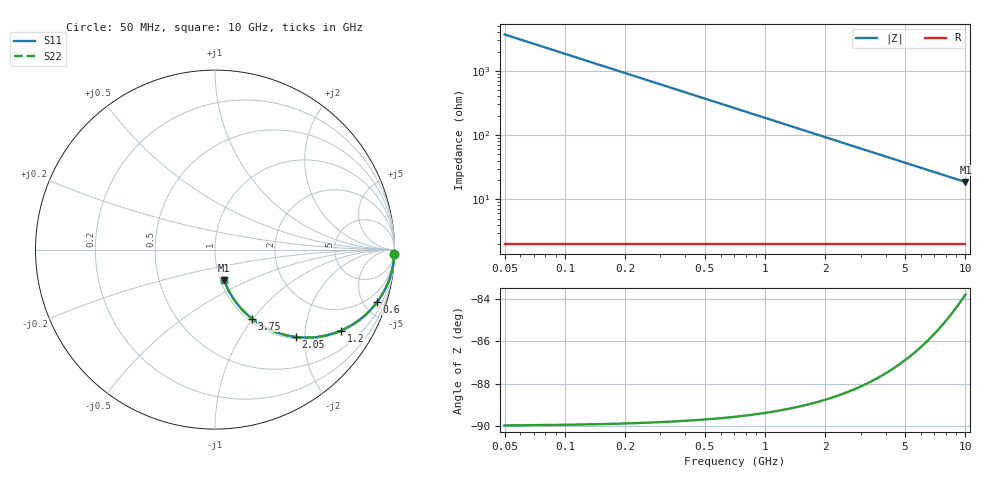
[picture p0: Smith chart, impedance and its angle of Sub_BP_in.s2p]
! Created Thu Jul 12 14:06:35 2018
# hz S ma R 50
! 2 Port Network Data from SP1.SP block
! freq  magS11  angS11  magS21  angS21  magS12  angS12  magS22  angS22
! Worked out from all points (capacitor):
!   200 points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, 50 MHz to 10 GHz, reference 50 ohm
!   read as one part in series: C = 861 fF near 100 MHz
!   lowest |Z| = 18.6 ohm at 10 GHz (marker M1)
!   S11 on the Smith chart (normalised r, x): 50 MHz: 1, -74; 600 MHz: 1.04, -6.16; 1.2 GHz: 1.04, -3.08; 2.05 GHz: 1.04, -1.80; 3.75 GHz: 1.04, -0.99; 10 GHz: 1.04, -0.37
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5e7  0.9996 -1.5  0.02704 88.4  0.02704 88.4  0.9996 -1.5
1e8  0.9985 -3.1  0.05403 86.8  0.05403 86.8  0.9985 -3.1
1.5e8  0.9966 -4.6  0.08089 85.3  0.08089 85.3  0.9966 -4.6
2e8  0.994 -6.2  0.1076 83.7  0.1076 83.7  0.994 -6.2
2.5e8  0.9906 -7.7  0.134 82.1  0.134 82.1  0.9906 -7.7
3.5e8  0.9819 -10.7  0.1859 79.1  0.1859 79.1  0.9819 -10.7
4.5e8  0.9705 -13.7  0.2363 76.1  0.2363 76.1  0.9705 -13.7
6e8  0.9493 -18.0  0.3082 71.7  0.3082 71.7  0.9493 -18.0
7e8  0.9328 -20.7  0.3533 68.9  0.3533 68.9  0.9328 -20.7
8.5e8  0.9053 -24.6  0.4164 64.9  0.4164 64.9  0.9053 -24.6
1e9  0.8755 -28.3  0.4737 61.1  0.4737 61.1  0.8755 -28.3
1.2e9  0.8338 -32.8  0.5413 56.5  0.5413 56.5  0.8338 -32.8
1.45e9  0.7808 -37.8  0.6125 51.3  0.6125 51.3  0.7808 -37.8
1.75e9  0.7194 -42.9  0.6811 46.0  0.6811 46.0  0.7194 -42.9
2.05e9  0.6624 -47.3  0.7345 41.5  0.7345 41.5  0.6624 -47.3
2.7e9  0.5574 -54.5  0.814 33.9  0.814 33.9  0.5574 -54.5
3.4e9  0.4706 -59.8  0.8651 28.0  0.8651 28.0  0.4706 -59.8
3.75e9  0.4354 -61.9  0.8827 25.8  0.8827 25.8  0.4354 -61.9
5.05e9  0.3382 -67.1  0.9227 19.7  0.9227 19.7  0.3382 -67.1
6.7e9  0.2617 -70.7  0.9463 15.1  0.9463 15.1  0.2617 -70.7
8.35e9  0.2129 -72.6  0.958 12.2  0.958 12.2  0.2129 -72.6
1e10  0.1793 -73.5  0.9646 10.3  0.9646 10.3  0.1793 -73.5
